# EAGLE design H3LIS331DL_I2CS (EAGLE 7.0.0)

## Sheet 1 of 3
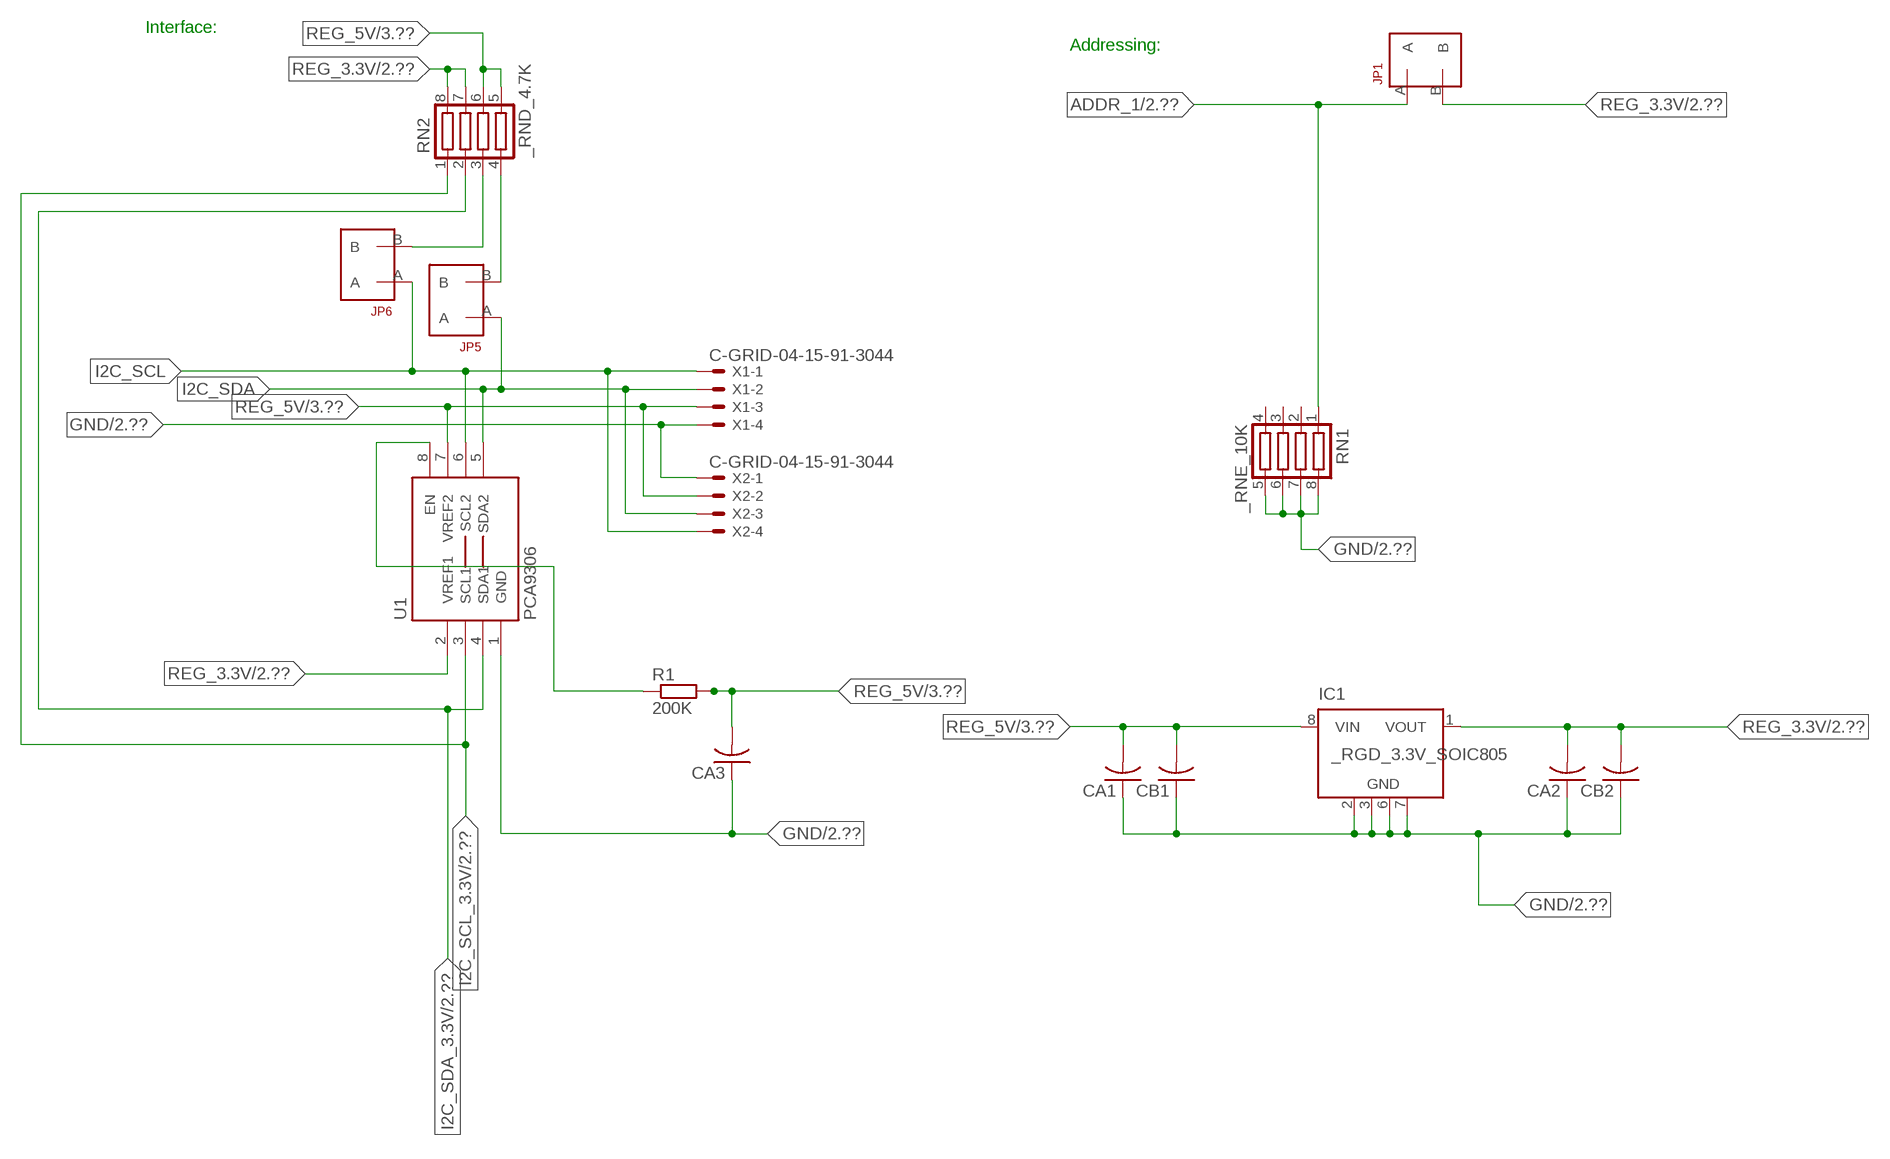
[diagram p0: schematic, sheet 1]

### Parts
CA1  CC1206KRX7R9BB104  [.1UF]
CA2  CC1206KRX7R9BB104  [.1UF]
CA3  CC1206KRX7R9BB104  [.1UF]
CB1  TMK316F106ZL-TC1206K  [TMK316F106ZL-T]
CB2  TMK316F106ZL-TC1206K  [TMK316F106ZL-T]
IC1  _RGD_3.3V_SOIC805  [_RGC_3.3V_SOIC8]
JP1  JUMPER_1X2_2MM  [JUMPER_1X2_2MM]
JP5  JUMPER_1X2_2MM  [JUMPER_1X2_2MM]
JP6  JUMPER_1X2_2MM  [JUMPER_1X2_2MM]
R1  200K  RESISTOR_SMT-0603  [R603]
RN1  _RNE_10K  [RNE]
RN2  _RND_4.7K  [RND]
U1  PCA9306  PCA9306_NCD  [PSOP-8]
X1  C-GRID-04-15-91-3044  [15-91-04]
X2  C-GRID-04-15-91-3044  [15-91-04]

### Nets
ADDR_1: JP1.A RN1.1 ; also sheet 2
GND: CA1.1 CA2.1 CA3.1 CB1.1 CB2.1 IC1.2(GND) IC1.3(GND) IC1.6(GND) IC1.7(GND) RN1.5 RN1.6 RN1.7 RN1.8 U1.1(GND) X1.4 X2.1 ; also sheet 2,3
I2C_SCL: JP6.A U1.6(SCL2) X1.1 X2.4
I2C_SCL_3.3V: RN2.1 U1.3(SCL1) ; also sheet 2
I2C_SDA: JP5.A U1.5(SDA2) X1.2 X2.3
I2C_SDA_3.3V: RN2.2 U1.4(SDA1) ; also sheet 2
N$1: JP6.B RN2.3
N$2: JP5.B RN2.4
N$3: R1.1 U1.8(EN)
REG_3.3V: CA2.2 CB2.2 IC1.1(VOUT) JP1.B RN2.7 RN2.8 U1.2(VREF1) ; also sheet 2
REG_5V: CA1.2 CA3.2 CB1.2 IC1.8(VIN) R1.2 RN2.5 RN2.6 U1.7(VREF2) X1.3 X2.2 ; also sheet 3
Unconnected: IC1.4(NC) IC1.5(NC) RN1.2 RN1.3 RN1.4

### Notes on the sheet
- Interface:
- Addressing:

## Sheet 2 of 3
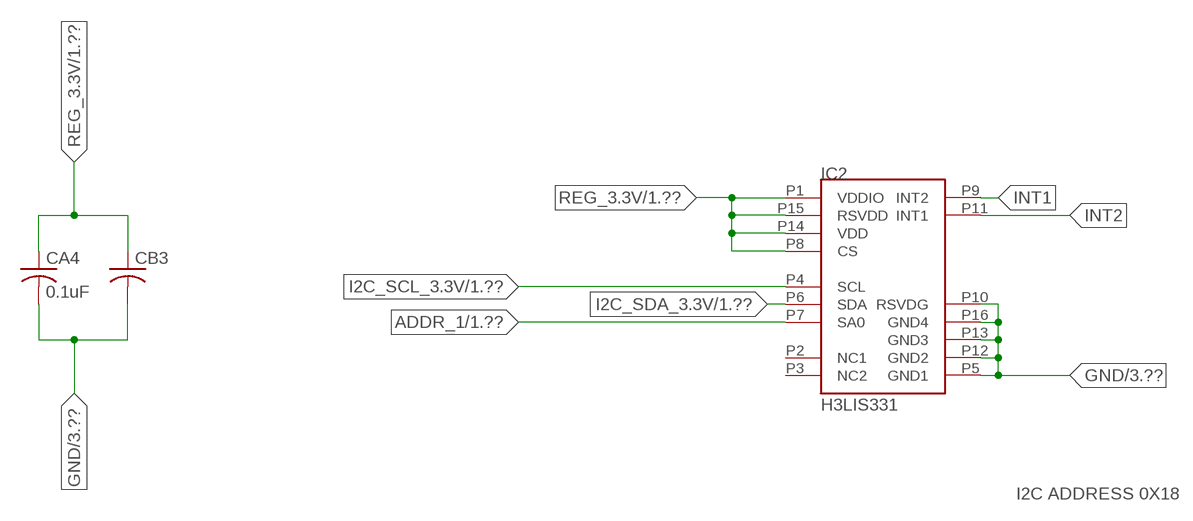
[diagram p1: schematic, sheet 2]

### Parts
CA4  0.1uF  CC1206KRX7R9BB104C1206K  [CC1206KRX7R9BB104]
CB3  _CB_10UF_25VC1206K  [_CB_10UF_25V]
IC2  H3LIS331  [LIS331]

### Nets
ADDR_1: IC2.P7(SA0) ; also sheet 1
GND: CA4.2 CB3.2 IC2.P5(GND1) IC2.P10(RSVDG) IC2.P12(GND2) IC2.P13(GND3) IC2.P16(GND4) ; also sheet 1,3
I2C_SCL_3.3V: IC2.P4(SCL) ; also sheet 1
I2C_SDA_3.3V: IC2.P6(SDA) ; also sheet 1
INT1: IC2.P9(INT2)
INT2: IC2.P11(INT1)
REG_3.3V: CA4.1 CB3.1 IC2.P1(VDDIO) IC2.P8(CS) IC2.P14(VDD) IC2.P15(RSVDD) ; also sheet 1
Unconnected: IC2.P2(NC1) IC2.P3(NC2)

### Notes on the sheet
- I2C ADDRESS 0X18

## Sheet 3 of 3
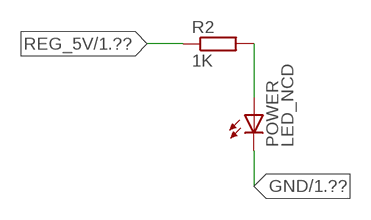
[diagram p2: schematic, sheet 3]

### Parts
POWER  LED_NCD  [CHIPLED_0603]
R2  1K  RESISTOR_SMT-0402  [R402]

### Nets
GND: POWER.C ; also sheet 1,2
N$4: POWER.A R2.2
REG_5V: R2.1 ; also sheet 1

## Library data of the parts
CA1-CA4 = NCD_ULTIMATE_LIBRARY:CC1206KRX7R9BB104: Capacitor CA .1uF 50V SMT C1206K CC1206KRX7R9BB104
CB1 CB2 = NCD_ULTIMATE_LIBRARY:TMK316F106ZL-T: Capacitor CB 10uF SMT 1206 TMK316F106ZL-T
CB3 = NCD_ULTIMATE_LIBRARY:_CB_10UF_25V: Capacitor 10uF SMT
IC1 = NCD_ULTIMATE_LIBRARY:_RGD_3.3V_SOIC8: Regulator Linear 3.3V Chip Positive VOLTAGE REGULATOR Digikey 497-1199-2-ND/L78L33ACD13TR
IC2 = NCD_ULTIMATE_AMAN:H3LIS331
JP1 JP5 JP6 = NCD_ULTIMATE_CONNECTORS:JUMPER_1X2_2MM
POWER = NCD_ULTIMATE_LIBRARY:LED_NCD: LED Digikey 754-1132-2-ND/APT2012SRCPRV
R1 R2 = NCD_ULTIMATE_LIBRARY:RESISTOR_SMT: NCD Resistor
RN1 = NCD_ULTIMATE_LIBRARY:_RNE_10K: Resistor Array RNE SMT 10K x 4 Single Resistor Source: http://www.ctscorp.com/components/Datasheets/CTSChipArrayDs.pdf Digikey 742C083103JPTR-ND/742C083103JP; OC_FARNELL: unknown; OC_NEWARK: unknown
RN2 = NCD_ULTIMATE_LIBRARY:_RND_4.7K: Resistor Array RND SMT 4.7K x 4 Single Resistor Source: http://www.ctscorp.com/components/Datasheets/CTSChipArrayDs.pdf Digikey 742C083472JPTR-ND/742C083472JP; OC_FARNELL: unknown; OC_NEWARK: unknown
U1 = NCD_ULTIMATE_LIBRARY:PCA9306_NCD: NCD Bidirectional I2C level shifter. NOT compatible with all available part number pinout schemes- DOUBLE CHECK!!!; PROD_ID: IC-10023
X1 X2 = NCD_ULTIMATE_CONNECTORS:C-GRID-04: CONNECTOR 4-Pos I2C wire to board 2.54 mm (0.100") pitch header Digikey WM1342-ND/0015912045; OC_FARNELL: unknown; OC_NEWARK: unknown

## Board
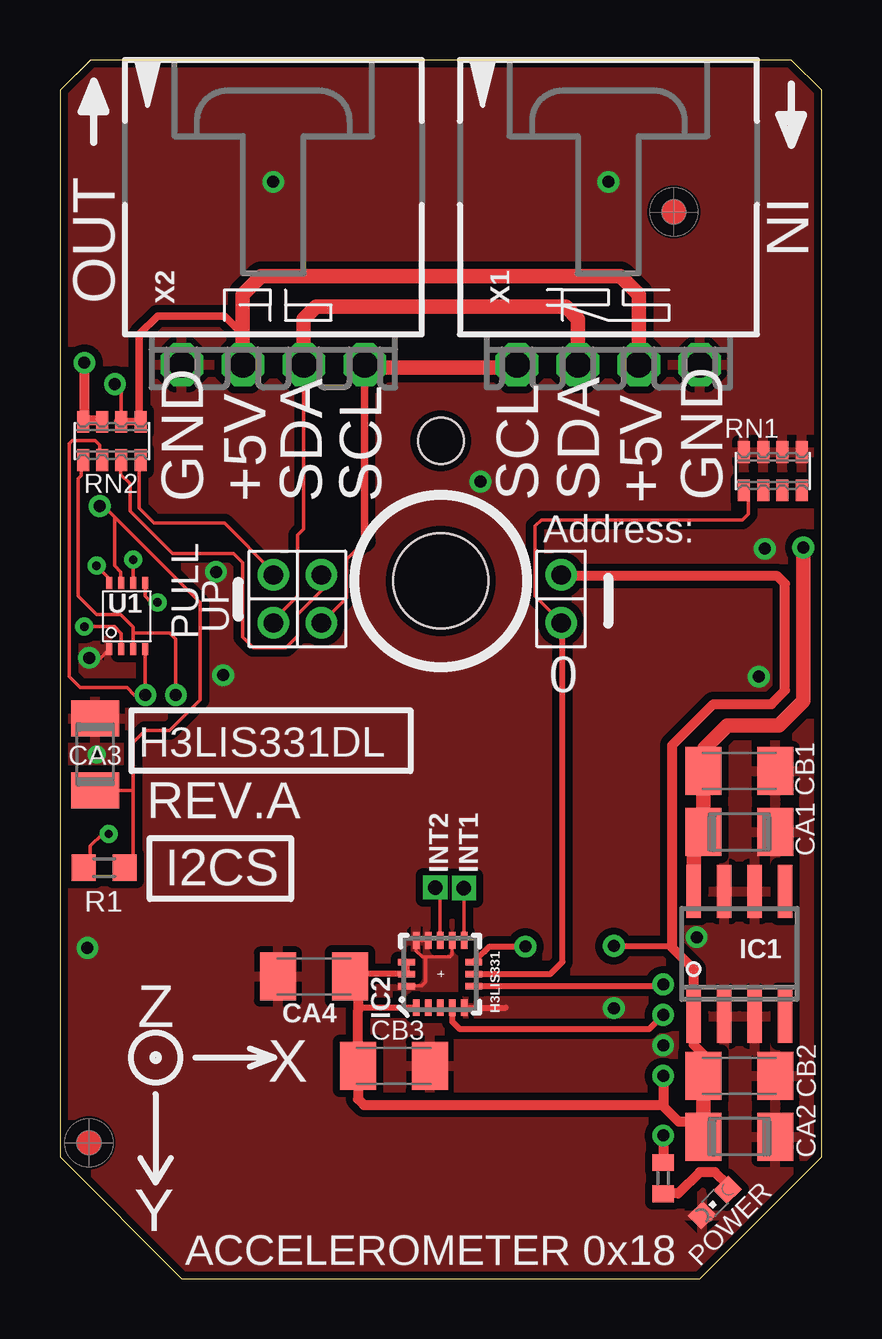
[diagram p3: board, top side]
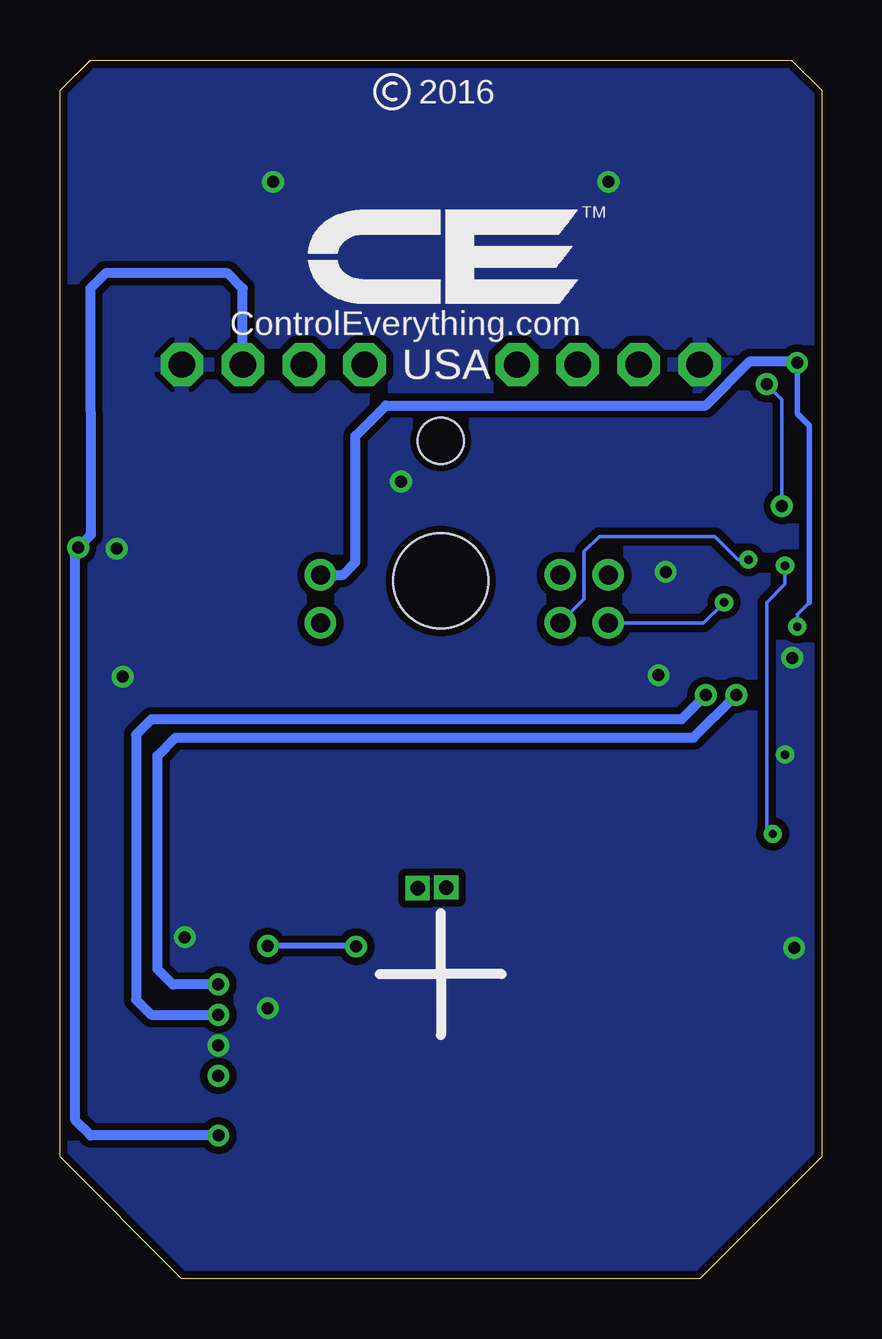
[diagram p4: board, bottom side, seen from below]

Size 31.75 x 50.8 mm. Coordinates in mm from the lower left corner, seen from the top.
Outline: 48 segments
Copper layers (1*16): Top 0.035mm / dielectric 1.5mm / Bottom 0.035mm
Design rules "default": minimum track width 5mil, minimum drill 24mil, track to track 5mil, track to pad 5mil, pad to pad 5mil, via to via 5mil, smd to smd 5mil, copper to edge 10mil, drill to drill 8mil, minimum pad ring 10mil, minimum via ring 8mil, stop-mask expansion 2mil, vias tented up to drill 0mil, thermal gap 10mil
Holes 3.96 mm at 15.88,29.08
Holes 1.91 mm at 15.88,34.93

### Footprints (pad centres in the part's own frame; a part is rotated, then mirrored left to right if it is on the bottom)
.1UF = smd 1.5 x 2: 1 -1.5,0; 2 1.5,0
CC1206KRX7R9BB104 = smd 1.5 x 2: 1 -1.5,0; 2 1.5,0
TMK316F106ZL-T = smd 1.5 x 2: 1 -1.5,0; 2 1.5,0
_CB_10UF_25V = smd 1.5 x 2: 1 -1.5,0; 2 1.5,0
_RGC_3.3V_SOIC8 = smd 0.6 x 2.2: 1 -1.905,-2.6; 2 -0.635,-2.6; 3 0.635,-2.6; 4 1.905,-2.6; 5 1.905,2.6; 6 0.635,2.6; 7 -0.635,2.6; 8 -1.905,2.6
LIS331 = smd 0.7 x 0.28: P1 -1.4,1; P2 -1.4,0.5; P3 -1.4,0; P4 -1.4,-0.5; P5 -1.4,-1; P9 1.4,-1; P10 1.4,-0.5; P11 1.4,0; P12 1.4,0.5; P13 1.4,1 | smd 0.28 x 0.7: P6 -0.5,-1.4; P7 0,-1.4; P8 0.5,-1.4; P14 0.5,1.4; P15 0,1.4; P16 -0.5,1.4
JUMPER_1X2_2MM = drill 0.8: A 0,2; B 0,0
CHIPLED_0603 = smd 0.8 x 0.876: A 0,-0.75; C 0,0.75
R603 = smd 1 x 1.1: 1 -0.85,0; 2 0.85,0
R402 = smd 0.7 x 0.9: 1 -0.65,0; 2 0.65,0
RNE = smd 0.5 x 0.9: 1 -1.2,-0.8; 2 -0.4,-0.8; 3 0.4,-0.8; 4 1.2,-0.8; 5 1.2,0.8; 6 0.4,0.8; 7 -0.4,0.8; 8 -1.2,0.8
RND = smd 0.5 x 0.9: 1 -1.2,-0.8; 2 -0.4,-0.8; 3 0.4,-0.8; 4 1.2,-0.8; 5 1.2,0.8; 6 0.4,0.8; 7 -0.4,0.8; 8 -1.2,0.8
PSOP-8 = smd 0.25 x 0.5: 1 -0.73,-1.37; 2 -0.23,-1.37; 3 0.27,-1.37; 4 0.77,-1.37; 5 0.77,1.38; 6 0.27,1.38; 7 -0.23,1.38; 8 -0.73,1.38
15-91-04 = drill 1.1 pad 1.778 octagon: 1 -3.81,-7.62; 2 -1.27,-7.62; 3 1.27,-7.62; 4 3.81,-7.62

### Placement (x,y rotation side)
CA1  28.32,18.62 180 top
CA2  28.32,5.92 180 top
CA3  1.46,21.86 270 top
CA4  10.59,12.6 180 top
CB1  28.32,21.16 180 top
CB2  28.32,8.46 180 top
CB3  13.92,8.86 0 top
IC1  28.32,13.54 0 top
IC2  15.85,12.7 90 top
JP1  20.89,29.34 180 top
JP5  8.89,29.34 180 top
JP6  10.9,29.34 180 top
POWER  27.3,3.18 135 top
R1  1.84,17.13 0 top
R2  25.15,4.19 270 top
RN1  29.72,33.66 0 top
RN2  2.16,34.93 0 top
U1  2.79,27.61 0 top
U$5  [VISION_REF10]  1.21,5.66 90 top
U$28  [VISION_REF10]  25.59,44.46 90 top
X1  22.86,45.72 0 top
X2  8.89,45.72 0 top

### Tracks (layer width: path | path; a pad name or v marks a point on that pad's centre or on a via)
ADDR_1
  Top 0.152: JP1.A 20.89,27.37 19.81,28.45 19.81,31.37 20.07,31.62 28.45,31.62 28.7,31.88 28.7,32.78 RN1.1
  Top 0.254: IC2.P7 20.45,12.7 20.95,13.21 20.95,27.28 JP1.A
GND  (via drill 0.35, 0.5)
  Top 0.152: CA3.1 1.52,23.42 1.52,23.62 | U1.1 1.7,25.88 v1.22,25.88 | IC2.P12 IC2.P13 14.85,13.68 15.11,13.41 15.24,13.41 | IC2.P10 16.35,13.51 16.26,13.41 15.24,13.41 | IC2.P16 15.07,12.2 15.24,12.37 15.24,13.41
  Top 0.254: IC2.P5 18.59,11.3
  other vias: 8.89,45.72 22.86,45.72 25.15,9.73 6.8,25.16 17.53,33.22 26.55,14.24 1.15,13.79 6.5,29.46 1.52,21.84 29.13,25.1 29.39,30.43 23.09,11.28
  pour Top (isolate 0.305): -1.27,0 -1.27,50.8 33.02,50.8 33.02,0
  pour Bottom (isolate 0.305): -5.08,0 -5.08,50.8 35.56,50.8 35.56,0
I2C_SCL  (via drill 0.35)
  Top 0.152: 12.7,30.73 11.94,29.97 11.94,28.38 JP6.A | v3.05,29.97 3.06,29.96 U1.6
  Top 0.305: 12.7,30.73 X2.4
  Top 0.406: X2.4 12.7,37.97 | 19.05,37.97 X1.1
  Top 0.61: 12.7,37.97 19.05,37.97
  Bottom 0.152: JP6.A 9.91,28.33 9.91,30.3 9.27,30.94 4.45,30.94 3.48,29.97 v3.05,29.97
I2C_SCL_3.3V  (via drill 0.5)
  Top 0.152: RN2.1 0.89,34.07 0.89,33.48 0.77,33.35 0.77,29.1 0.76,29.09 0.76,28.45 1.52,27.69 2.54,27.69 3.06,27.17 3.06,26.92 | 3.06,26.92 U1.3 | v4.83,24.33 v4.83,24.34 4.83,26.67 4.57,26.92 3.06,26.92
  Top 0.254: v25.15,11 24.56,10.41 16.66,10.41 16.35,10.73 IC2.P4
  Bottom 0.406: v4.83,24.33 5.84,23.32 27.94,23.32 28.58,22.68 28.58,11.63 27.94,11 v25.15,11
I2C_SDA  (via drill 0.35)
  Top 0.152: JP5.A 8.89,27.44 9.91,28.45 9.91,30.99 10.16,31.24 10.16,34.92 X2.3 | U1.5 3.56,28.45 3.81,28.19 v4.06,28.19
  Top 0.61: X2.3 10.16,40.01 10.67,40.51 21.09,40.51 21.59,40.01 X1.2
  Bottom 0.152: v4.06,28.19 4.92,27.34 JP5.A
I2C_SDA_3.3V  (via drill 0.5)
  Top 0.152: RN2.2 1.65,34.14 1.65,34.75 1.46,34.94 0.51,34.94 0.38,34.81 0.38,26.37 0.38,26.36 0.38,25.1 0.84,24.64 2.79,24.64 3.1,24.33 v3.56,24.33 v3.56,24.34 U1.4
  Top 0.254: IC2.P6 25.08,12.2 v25.15,12.27
  Bottom 0.406: v25.15,12.27 27.05,12.27 27.69,12.9 27.69,21.79 26.93,22.56 5.34,22.56 v3.56,24.33
INT1  (via drill 0.6)
  Top 0.152: IC2.P9 v16.85,16.27 v16.84,16.28
INT2  (via drill 0.6)
  Top 0.152: IC2.P11 15.85,16.1 v15.65,16.31
N$1
  Top 0.152: JP6.B 10.92,29.31 10.92,28.7 9.91,27.69 9.91,26.8 9.42,26.31 8.06,26.31 7.62,26.75 7.62,29.84 7.24,30.23 4.7,30.23 2.92,32 2.92,33.15 2.54,33.53 2.54,34.1 RN2.3
  Top 0.305: 2.54,34.02 RN2.3
N$2
  Top 0.152: JP5.B 8.89,29.46 6.86,31.5 3.94,31.5 3.3,32.13 3.3,34.07 RN2.4
  Top 0.305: 3.37,33.88 RN2.4
N$3  (via drill 0.35)
  Top 0.152: R1.1 1.27,17.41 1.27,18.03 1.78,18.54 v2.03,18.54 | v1.52,29.72 2.06,29.18 U1.8
  Bottom 0.152: v2.03,18.54 2.29,18.8 2.29,28.19 1.52,28.96 v1.52,29.72
N$4
  Top 0.406: POWER.A 27.84,3.92 27.3,4.45 26.67,4.45 25.78,3.56 25.16,3.56 R2.2
REG_3.3V  (via drill 0.35, 0.5)
  Top 0.152: v1.02,27.18 2.29,27.18 2.56,26.9 U1.2
  Top 0.254: IC2.P14 IC2.P15 12.42,12.7 12.42,12.09 | IC2.P8 17.69,13.64 17.7,13.64 17.91,13.84 v19.41,13.84 | v23.09,13.87 25.53,13.87 25.53,13.95 | IC2.P1 12.42,11.3 12.42,11.15
  Top 0.406: CB2.2 26.82,9.35 26.42,9.75 26.42,10.36 | v25.15,8.46 25.15,7.19 | 25.15,7.19 25.78,6.55 26.82,6.55 | IC1.1 26.42,12.9 25.53,13.79 25.53,13.95 25.53,22.24 27.24,23.95 29.66,23.95 30.23,24.52 30.23,28.97 29.91,29.29 20.95,29.29 JP1.B | 26.52,5.62 CA2.2 | v1.02,38.18 1.02,35.78 | 1.02,35.78 RN2.8 | 1.02,35.78 1.71,35.78 RN2.7 | CA4.1 12.42,12.6 12.42,12.09 12.42,11.15 CB3.1 12.42,7.49 12.68,7.24 25.1,7.24 25.15,7.19
  Top 0.61: CB2.2 26.82,6.55 CA2.2 | 26.42,10.36 IC1.1
  Bottom 0.152: 0.51,28.19 1.02,27.69 v1.02,27.18
  Bottom 0.229: 0.51,28.19 0.51,35.56 1.02,36.07 v1.02,38.18
  Bottom 0.254: v19.41,13.84 19.43,13.87 v23.09,13.87
  Bottom 0.406: v1.02,38.18 1.08,38.24 2.99,38.24 4.83,36.4 18.16,36.4 19.43,35.13 19.43,29.87 19.94,29.34 JP1.B
REG_5V  (via drill 0.5)
  Top 0.152: RN2.6 2.56,37.01 v2.29,37.29 | R1.2 3.05,17.49 3.05,20.36 | 3.05,20.36 3.05,22.35 3.56,22.86 4.57,22.86 5.84,24.13 5.84,28.19 2.29,31.75 | CA3.2 3.05,20.36 | 2.29,31.75 1.83,32.21 v1.65,32.21 | U1.7 2.54,29.01 2.54,29.46 2.29,29.72 2.29,31.75
  Top 0.305: 7.62,39.37 7.5,39.37 | 2.42,35.74 RN2.6 RN2.5 3.31,35.8 3.31,39.37 4.07,40.13 6.86,40.13 7.62,39.37 | X2.2 7.62,39.37
  Top 0.406: v25.15,5.97 R2.1
  Top 0.61: X1.3 24.13,41.02 23.37,41.78 8.38,41.78 7.62,41.02 X2.2 | IC1.8 26.42,18.21 CA1.2 CB1.2 26.86,21.2 26.86,22.11 27.82,23.06 29.98,23.06 30.99,24.08 v30.99,30.48
  Bottom 0.152: v1.65,32.21 1.65,36.65 v2.29,37.29
  Bottom 0.406: X1.3 24.13,41.28 24.77,41.91 29.84,41.91 30.48,41.27 30.47,31 v30.99,30.48 31.11,30.36 31.11,6.6 30.48,5.97 v25.15,5.97

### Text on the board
tNames: IN | OUT | GND | +5V | SDA | SCL | SCL | SDA | +5V | GND | Address: | PULL | UP | 0 | H3LIS331DL | REV.A | INT2 | INT1 | I2CS | Z | X | Y | ACCELEROMETER 0x18
bNames: 2016 | TM | ControlEverything.com | USA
